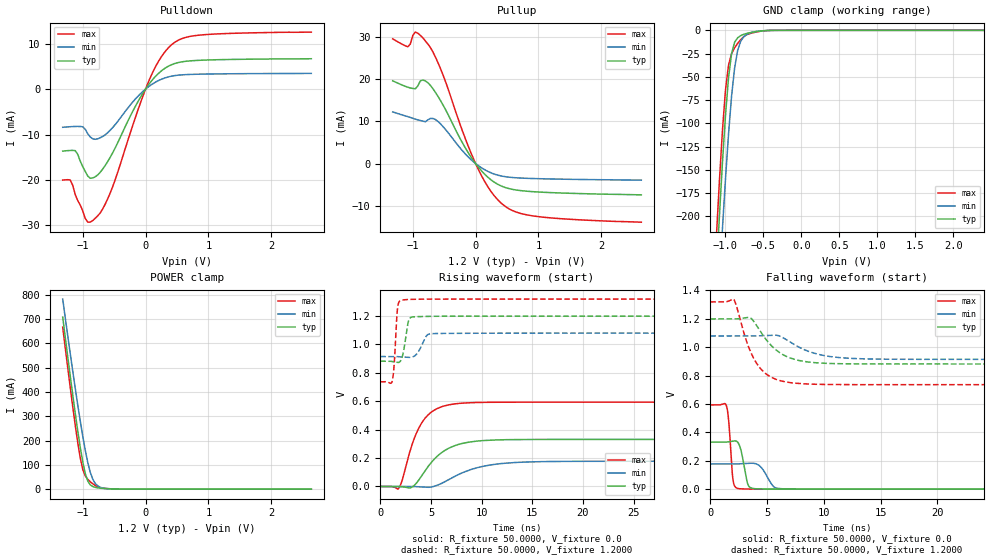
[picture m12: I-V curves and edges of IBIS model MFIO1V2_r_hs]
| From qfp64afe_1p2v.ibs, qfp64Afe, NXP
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[Model] MFIO1V2_r_hs
|   Model MFIO1V2_r_hs
| This model was characterised for following simulation conditions:
| External (pad) voltage:
|   - Typ: 1.2V,   - Min: 1.08V,   - Max: 1.32V
| Library cells for typ/min/max conditions are connected as defined below:
|  IO - External Pad
|  A - Core Input
|  EN - Output Buffer Enable
|  BOOST - vdde
|  EHS - vdd
|  ENZI - vdd
|  EPD - vdd
|  EPUN - gnd
|  ZI - NC
|  ZIF - NC
|  gnd - gnd
|  gnde - gnde
|  vdd - vdd
|  vdde - vdde
| All other pins connected to ground
Model_type I/O
Polarity   Non-Inverting
Enable   Active-Low
Vinl =   0.3600V
Vinh =   0.8400V
Vmeas =  0.6000V
Cref =   20.0000F
Rref =   1.0000M
Vref =   0.0V
C_comp   1.6368pF   1.5495pF   1.7159pF
|C_comp_pullup   0.8309pF   0.8676pF   0.7830pF
|C_comp_pulldown   0.5929pF   0.6311pF   0.5574pF
[Model Spec]
| variable   typ   min   max
Vinh   0.3600V   0.3240V   0.3960V
Vinl   0.8400V   0.7560V   0.9240V
Vmeas   0.6000V   0.5400V   0.6600V
[Temperature Range]   25.0000   0.1250k   -40.0000
[Voltage Range]   1.2000V   1.0800V   1.3200V
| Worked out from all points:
|   slope of the pulldown table from 0 to 0.18 V, typ, clamps not added: 58.2 ohm
|   slope of the pullup table from 0 to 0.18 V, typ, clamps not added: 59.4 ohm
|   GND clamp passes 1 mA (typ) near -0.56 V on its own axis
|   POWER clamp passes 1 mA (typ) near -0.54 V on its own axis
|   rising waveform, R_fixture 50.0000, V_fixture 0.0: 20-80 % time 2.65ns typ, 3.73ns min, 1.92ns max; typ from 0 V to 0.331 V
|   rising waveform, R_fixture 50.0000, V_fixture 1.2000: 20-80 % time 420ps typ, 689ps min, 271ps max; typ from 0.882 V to 1.2 V
|   falling waveform, R_fixture 50.0000, V_fixture 0.0: 20-80 % time 471ps typ, 797ps min, 303ps max; typ from 0.331 V to 0 V
|   falling waveform, R_fixture 50.0000, V_fixture 1.2000: 20-80 % time 2.23ns typ, 2.81ns min, 1.78ns max; typ from 1.2 V to 0.882 V
[Pulldown]
|Voltage   I(typ)   I(min)   I(max)
-1.32V    -13.65mA   -8.413mA   -20.02mA
-1.2V     -13.51mA   -8.286mA   -20.01mA
-1.12V    -13.55mA   -8.228mA   -23.23mA
-920mV    -19.16mA   -9.85mA    -29.29mA
-720mV    -18.27mA   -10.7mA    -27.21mA
-520mV    -13.92mA   -8.406mA   -21.33mA
-160mV    -3.727mA   -2.148mA   -6.154mA
80mV      1.535mA    840.4uA    2.681mA
280mV     4.299mA    2.312mA    7.674mA
480mV     5.684mA    2.989mA    10.42mA
960mV     6.383mA    3.3mA      11.99mA
2.64V     6.67mA     3.446mA    12.53mA
[Pullup]
|Voltage   I(typ)   I(min)   I(max)
-1.32V    19.64mA    12.26mA    29.6mA
-1.08V    18.12mA    11.13mA    27.73mA
-960mV    17.74mA    10.54mA    31.21mA
-840mV    19.83mA    10.07mA    29.84mA
-720mV    18.57mA    10.71mA    27.56mA
-520mV    13.94mA    8.794mA    21.09mA
-200mV    4.663mA    2.883mA    7.362mA
40mV      -771.3uA   -452.7uA   -1.28mA
240mV     -3.804mA   -2.171mA   -6.507mA
480mV     -5.732mA   -3.143mA   -10.26mA
1.04V     -6.794mA   -3.614mA   -12.68mA
2.64V     -7.439mA   -3.951mA   -13.93mA
[GND_clamp]
|Voltage   I(typ)   I(min)   I(max)
-1.32V    -596.2mA   -647.7mA   -564.2mA
-1.12V    -261.7mA   -329.6mA   -222.8mA
-1.08V    -200.1mA   -270.2mA   -162.2mA
-1.04V    -142.4mA   -213.4mA   -108mA
-1V       -91.66mA   -160.1mA   -64.4mA
-960mV    -51.26mA   -111.8mA   -37.36mA
-920mV    -25.17mA   -71.04mA   -25.19mA
-880mV    -12.89mA   -40.68mA   -18.85mA
-800mV    -5.7mA     -11.79mA   -10.05mA
-680mV    -2.586mA   -2.926mA   -3.538mA
-440mV    -160.8uA   -186.1uA   -197.3uA
2.64V     0A         0A         0A
[POWER_clamp]
|Voltage   I(typ)   I(min)   I(max)
-1.32V    708.1mA    782.2mA    666.5mA
-1.2V     465.5mA    558mA      418.6mA
-1.12V    311.6mA    414.8mA    262.8mA
-1.04V    171.5mA    279.6mA    128.1mA
-1V       111.7mA    217mA      80.3mA
-960mV    64.07mA    159.3mA    53.87mA
-920mV    33.02mA    108.9mA    40.24mA
-880mV    17.44mA    68.44mA    30.42mA
-840mV    10.78mA    40.19mA    22.06mA
-760mV    5.295mA    13.21mA    9.362mA
-440mV    235.7uA    303.1uA    277.6uA
2.64V     0A         0A         0A
[Ramp]
| variable   typ   min   max
dV/dt_r  0.1989/2.6495n   0.1066/3.7245n   0.3561/1.9166n
dV/dt_f  0.1904/2.2322n   98.8032m/2.8094n   0.3496/1.7781n
R_load = 50.0000
[Rising Waveform]
R_fixture= 50.0000
V_fixture= 0.0
V_fixture_min= 0.0
V_fixture_max= 0.0
|time   V(typ)   V(min)   V(max)
0s        1.234nV    117.7nV    49.88pV
1.836ns   -139.8uV   80.48uV    -11.1mV
2.916ns   -10.79mV   -3.985uV   244.6mV
3.442ns   13.72mV    -873.6uV   355.1mV
4.708ns   139.9mV    -5.514mV   503.3mV
6.165ns   244mV      26.22mV    564mV
8.03ns    302.1mV    94.36mV    586.5mV
11.39ns   327.6mV    157mV      593.1mV
16.39ns   331.4mV    175.6mV    593.6mV
100ns     331.4mV    177.7mV    593.5mV
[Rising Waveform]
R_fixture= 50.0000
V_fixture= 1.2000
V_fixture_min= 1.0800
V_fixture_max= 1.3200
|time   V(typ)   V(min)   V(max)
0s        882mV      914.8mV    736.7mV
1.163ns   880.1mV    915mV      738.3mV
1.362ns   877.5mV    915.2mV    848.4mV
1.739ns   872.7mV    913.9mV    1.274V
2.144ns   908.4mV    912mV      1.312V
2.493ns   1.039V     910.2mV    1.315V
2.957ns   1.188V     908.9mV    1.317V
4.607ns   1.198V     1.064V     1.319V
5.502ns   1.198V     1.077V     1.319V
100ns     1.199V     1.079V     1.319V
[Falling Waveform]
R_fixture= 50.0000
V_fixture= 0.0
V_fixture_min= 0.0
V_fixture_max= 0.0
|time   V(typ)   V(min)   V(max)
0s        331.4mV    177.7mV    593.5mV
1.422ns   331.9mV    177.7mV    587.4mV
1.621ns   333.8mV    177.6mV    481.2mV
2.017ns   338.9mV    177.5mV    56.5mV
2.612ns   298.8mV    178.8mV    2.701mV
3.324ns   31.08mV    182mV      996.4uV
4.117ns   2.211mV    176mV      450.6uV
5.606ns   575uV      15.88mV    122.8uV
6.717ns   262.3uV    1.618mV    49.44uV
100ns     2.826nV    122.2nV    7.762nV
[Falling Waveform]
R_fixture= 50.0000
V_fixture= 1.2000
V_fixture_min= 1.0800
V_fixture_max= 1.3200
|time   V(typ)   V(min)   V(max)
0s        1.199V     1.079V     1.319V
2.058ns   1.199V     1.079V     1.338V
2.284ns   1.2V       1.079V     1.296V
3.455ns   1.21V      1.079V     985.8mV
4.238ns   1.134V     1.08V      867.9mV
5.656ns   989.5mV    1.086V     778mV
7.732ns   908.3mV    1.004V     744.9mV
10.56ns   885.7mV    934.4mV    737.5mV
14.62ns   882.3mV    916.5mV    736.7mV
100ns     882mV      914.8mV    736.7mV
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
